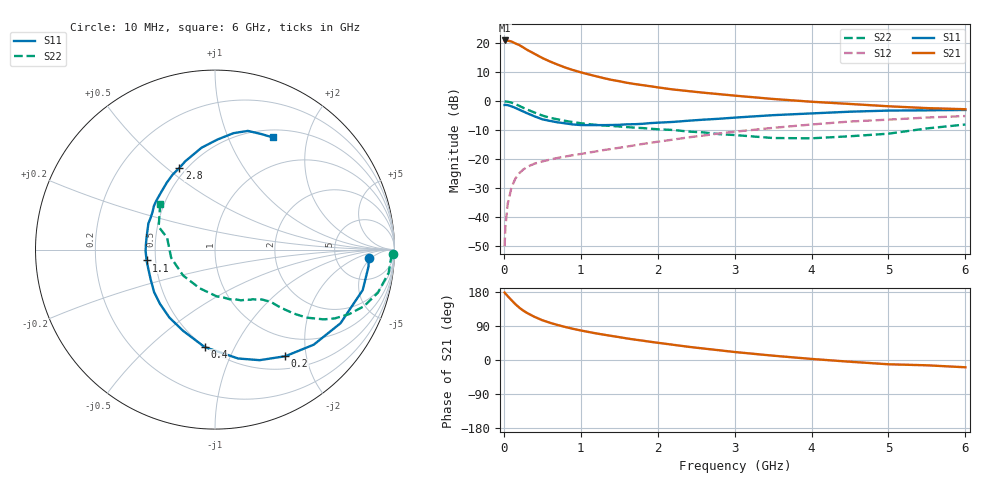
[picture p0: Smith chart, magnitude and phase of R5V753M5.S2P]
! SIEMENS Small Signal Semiconductors
! BFR183
! Si NPN RF Bipolar Junction Transistor in SOT23
! VCE = 0.75 V  IC = 3.5 mA
! Common Emitter S-Parameters:  May  1996
# GHz  S  MA  R  50
!  f  S11  S21  S12  S22
! GHz  MAG  ANG  MAG  ANG  MAG  ANG  MAG  ANG
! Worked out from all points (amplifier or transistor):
!   36 points, 10 MHz to 6 GHz, reference 50 ohm
!   highest |S21| = 20.8 dB at 10 MHz (marker M1)
!   |S21| within 3 dB of that: start of sweep to 288.7 MHz
!   unconditionally stable (mu >= 1): 1.106 GHz to 3.111 GHz
!   at 250 MHz: K = 0.34, MSG = 21.0 dB, |S12| = -23.6 dB
!   at 1.4 GHz: K = 1.08, MAG = 10.1 dB, |S12| = -16.5 dB
!   at 6 GHz: K = 0.95, MSG = 1.2 dB, |S12| = -5.1 dB
!   S11 on the Smith chart (normalised r, x): 10 MHz: 12, -4; 200 MHz: 0.68, -1.64; 400 MHz: 0.50, -0.77; 1.1 GHz: 0.45, -0.06; 2.8 GHz: 0.46, +0.55; 6 GHz: 0.60, +1.47
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0.01  0.8565 -3.1  11.02 178.0  0.0032 90.3  0.9895 -1.5
0.02  0.8606 -6.2  10.89 175.4  0.0069 88.4  0.9818 -3.0
0.05  0.8533 -15.3  10.96 168.6  0.017 82.3  0.9762 -7.6
0.1  0.8108 -30.4  10.58 157.8  0.0329 74.3  0.939 -14.8
0.15  0.7638 -43.9  9.804 147.2  0.0465 67.8  0.8882 -20.8
0.2  0.7115 -56.6  9.197 138.4  0.0573 62.0  0.8281 -25.8
0.25  0.6644 -68.0  8.4 130.7  0.0662 57.5  0.7692 -29.9
0.3  0.6203 -78.0  7.639 124.3  0.0735 54.6  0.7196 -32.7
0.4  0.5459 -96.1  6.492 113.8  0.0841 50.1  0.6338 -36.7
0.5  0.4864 -111.4  5.505 105.0  0.0916 47.5  0.564 -39.1
0.6  0.4559 -123.9  4.79 98.2  0.0986 46.5  0.5166 -40.5
0.7  0.4308 -135.3  4.23 92.3  0.1053 46.0  0.4847 -41.5
0.9  0.396 -154.5  3.414 82.2  0.1176 46.4  0.4339 -42.9
1.1  0.3861 -171.0  2.883 74.0  0.1295 47.5  0.4025 -45.0
1.3  0.386 175.8  2.478 66.8  0.1439 48.2  0.38 -46.9
1.6  0.3988 158.5  2.063 56.9  0.165 49.0  0.3571 -51.1
2.2  0.438 133.4  1.584 40.2  0.2174 48.6  0.3185 -62.7
2.8  0.4967 113.5  1.315 25.7  0.2775 44.9  0.2706 -80.2
3.5  0.5726 97.5  1.087 11.4  0.3462 37.5  0.2316 -111.9
4.5  0.6568 81.0  0.892 -4.6  0.445 24.9  0.2484 -169.3
5.5  0.6936 68.1  0.757 -14.0  0.521 12.6  0.3388 157.9
6  0.7032 62.7  0.724 -19.2  0.5528 4.5  0.3956 140.5
